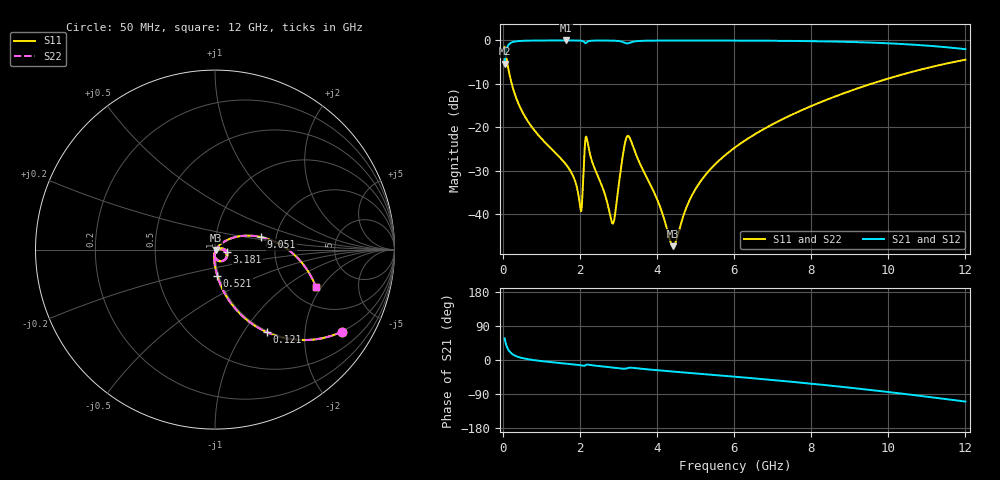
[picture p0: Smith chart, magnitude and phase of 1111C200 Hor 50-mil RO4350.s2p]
# GHz S MA R 50
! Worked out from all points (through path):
!   11951 points, 50 MHz to 12 GHz, reference 50 ohm
!   highest |S21| = -0.02 dB at 1.634 GHz (marker M1); lowest = -5.4 dB at 50 MHz (marker M2)
!   group delay of S21, straight-line fit = 26.5 ps
!   lowest |S11| = -47.4 dB at 4.42 GHz (marker M3), VSWR 1.01, Z = 50.4 - j0.198 ohm
!   |S11| at or under -10 dB: 234.4 MHz to 9.562 GHz (9.328 GHz wide, 190 % of centre)
!   |S22| runs from -47.4 to -1.5 dB; largest |S21 - S12| = 0
!   S11 on the Smith chart (normalised r, x): 50 MHz: 0.98, -3.10; 121 MHz: 0.98, -1.28; 521 MHz: 0.98, -0.29; 3.181 GHz: 1.14, -0.03; 9.051 GHz: 1.66, +0.25; 12 GHz: 2.72, -1.77
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0.05  0.8429 -32.9  0.538 57.1  0.538 57.1  0.8429 -32.9
0.121  0.5431 -57.9  0.8393 32.0  0.8393 32.0  0.5431 -57.9
0.244  0.305 -73.9  0.9519 16.0  0.9519 16.0  0.305 -73.9
0.521  0.1471 -85.0  0.9884 4.8  0.9884 4.8  0.1471 -85.0
1.634  0.03758 -97.3  0.9978 -9.4  0.9978 -9.4  0.03758 -97.3
1.859  0.02532 -96.4  0.9973 -11.7  0.9973 -11.7  0.02532 -96.4
2.001  0.01279 -74.7  0.9937 -13.5  0.9937 -13.5  0.01279 -74.7
2.042  0.01115 -34.1  0.9894 -14.2  0.9894 -14.2  0.01115 -34.1
2.137  0.0661 -19.3  0.934 -14.7  0.934 -14.7  0.0661 -19.3
2.187  0.07248 -65.2  0.9547 -12.1  0.9547 -12.1  0.07248 -65.2
2.863  0.007774 -35.3  0.9923 -19.9  0.9923 -19.9  0.007774 -35.3
2.92  0.01031 -3.4  0.99 -20.6  0.99 -20.6  0.01031 -3.4
3.181  0.06864 -12.4  0.9322 -22.9  0.9322 -22.9  0.06864 -12.4
3.3  0.07444 -58.2  0.9399 -20.4  0.9399 -20.4  0.07444 -58.2
4.034  0.01374 -93.9  0.9942 -27.2  0.9942 -27.2  0.01374 -93.9
4.42  0.004262 -27.5  0.9955 -30.5  0.9955 -30.5  0.004262 -27.5
5.042  0.02074 44.0  0.9958 -35.7  0.9958 -35.7  0.02074 44.0
6.025  0.05845 42.3  0.9943 -44.1  0.9943 -44.1  0.05845 42.3
8.017  0.1763 25.9  0.9794 -62.6  0.9794 -62.6  0.1763 25.9
9.051  0.2651 15.3  0.9586 -73.6  0.9586 -73.6  0.2651 15.3
10.009  0.3644 4.5  0.9249 -84.6  0.9249 -84.6  0.3644 4.5
12  0.5994 -20.3  0.7926 -109.6  0.7926 -109.6  0.5994 -20.3
